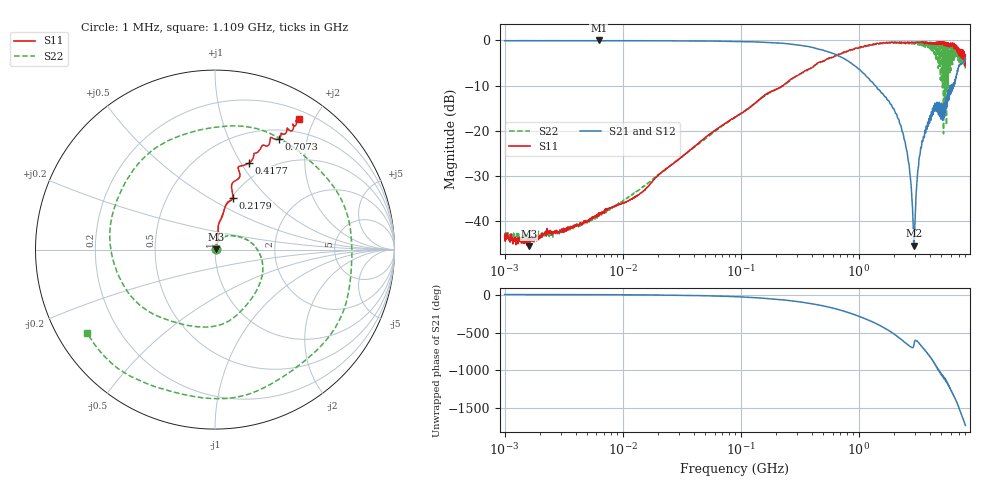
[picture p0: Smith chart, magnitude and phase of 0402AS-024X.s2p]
!s-Parameter Generated by FASTRON Sdn. Bhd.
!FASTRON P/N : 0402AS-024X
!Keysight Technologies: E5071C_MY46733604_B.14.02
!Date: Mon Dec 01 10:33:37 2025
!Version  :Rev00  Mon Dec 01 10:33:37 2025
!Data & Calibration Information:
!Freq  S11:SOLT2(ON)  S21:SOLT2(ON)  S12:SOLT2(ON)  S22:SOLT2(ON)
!PortZ  Port1:50+j0  Port2:50+j0
!When reading reference impedance value at option line is always used.
! Remarks : This data is being provided solely for informational purposes.
# Hz S dB R 50
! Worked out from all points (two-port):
!   1601 points, 1 MHz to 8 GHz, reference 50 ohm
!   highest |S21| = -0.01 dB at 6.268 MHz (marker M1); lowest = -45.5 dB at 2.927 GHz (marker M2)
!   |S21| within 3 dB of the highest: start of sweep to 624.6 MHz
!   lowest |S11| = -45.6 dB at 1.605 MHz (marker M3), VSWR 1.01, Z = 50.5 + j0.256 ohm
!   |S11| at or under -10 dB: start of sweep to 228.1 MHz
!   |S22| runs from -44.7 to -0.2 dB; largest |S21 - S12| = 0.021
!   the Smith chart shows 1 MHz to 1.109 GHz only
!   S11 on the Smith chart (normalised r, x): 1 MHz: 1.01, +0.01; 217.9 MHz: 1.01, +0.64; 417.7 MHz: 0.82, +1.09; 707.3 MHz: 0.62, +1.55; 1.109 GHz: 0.31, +1.79
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1000000  -43.40 24.1  -0.07 -0.3  -0.05 -0.4  -43.00 18.1
1604653  -45.60 28.9  -0.05 -0.6  -0.04 -0.5  -43.80 13.7
4479405  -40.60 52.1  -0.07 -1.5  -0.06 -1.4  -40.80 51.9
6268472  -38.20 52.1  -0.01 -1.7  -0.17 -1.6  -39.00 56.7
2.00676e7  -29.80 70.9  -0.08 -6.5  -0.08 -6.4  -29.80 69.5
8.994653e7  -17.00 81.9  -0.21 -28.3  -0.21 -28.3  -17.10 32.0
2.179466e8  -10.30 71.3  -0.60 -67.1  -0.60 -67.1  -10.40 -31.1
4.006501e8  -6.06 70.9  -1.52 -122.0  -1.51 -122.0  -5.93 -137.0
4.177449e8  -5.70 68.5  -1.64 -127.0  -1.63 -127.0  -5.62 -145.0
7.072899e8  -2.97 60.1  -3.66 152.0  -3.65 152.0  -2.90 62.8
1.108954e9  -1.28 57.3  -7.38 46.9  -7.37 46.8  -1.40 -147.0
1.365017e9  -0.89 61.5  -9.93 -14.1  -9.94 -14.1  -0.81 86.6
1.558366e9  -0.66 66.1  -11.60 -58.6  -11.60 -58.7  -0.59 -7.0
1.7949e9  -0.45 71.4  -13.40 -114.0  -13.40 -114.0  -0.62 -123.0
2.071864e9  -0.49 76.9  -16.20 -179.0  -16.20 -179.0  -0.54 101.0
2.44288e9  -0.58 82.2  -22.20 94.5  -22.10 94.4  -0.41 -81.3
2.662964e9  -0.54 88.3  -27.40 47.8  -27.40 47.6  -0.69 172.0
2.927065e9  -0.51 94.9  -45.50 55.3  -45.60 55.5  -0.36 47.3
3.183204e9  -0.39 101.0  -28.40 89.6  -28.40 89.1  -0.69 -89.3
3.548043e9  -0.39 111.0  -21.30 3.3  -21.20 2.9  -1.31 82.4
3.933151e9  -0.65 116.0  -17.30 -81.7  -17.30 -82.1  -1.63 -92.2
8e9  -3.15 -113.0  -4.08 76.3  -4.12 76.0  -6.35 106.0
